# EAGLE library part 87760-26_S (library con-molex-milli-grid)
HEADER
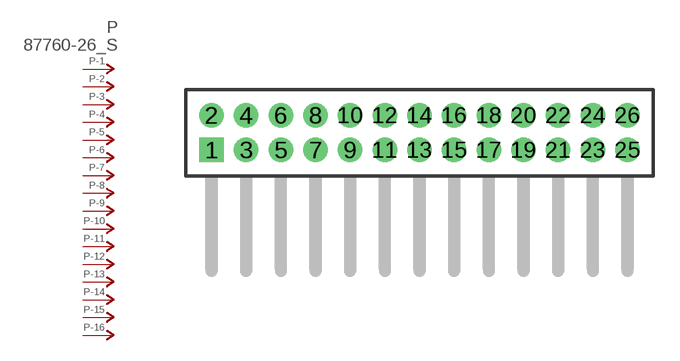
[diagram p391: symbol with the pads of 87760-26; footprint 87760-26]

Designator prefix P; gates -1=P-NV -2=P-N -3=P-N -4=P-N -5=P-N -6=P-N -7=P-N -8=P-N -9=P-N -10=P-N -11=P-N -12=P-N -13=P-N -14=P-N -15=P-N -16=P-N -17=P-N -18=P-N -19=P-N -20=P-N -21=P-N -22=P-N -23=P-N -24=P-N -25=P-N -26=P-N

## 87760-26_S  [87760-26]
1  -1:P  pas
2  -2:P  pas
3  -3:P  pas
4  -4:P  pas
5  -5:P  pas
6  -6:P  pas
7  -7:P  pas
8  -8:P  pas
9  -9:P  pas
10  -10:P  pas
11  -11:P  pas
12  -12:P  pas
13  -13:P  pas
14  -14:P  pas
15  -15:P  pas
16  -16:P  pas
17  -17:P  pas
18  -18:P  pas
19  -19:P  pas
20  -20:P  pas
21  -21:P  pas
22  -22:P  pas
23  -23:P  pas
24  -24:P  pas
25  -25:P  pas
26  -26:P  pas

## Footprint 87760-26 (pad centres in mm)
HEADER Dual Row, Right Angle
drill 0.914 square: 1 -12,-1
drill 0.914: 2 -12,1; 3 -10,-1; 4 -10,1; 5 -8,-1; 6 -8,1; 7 -6,-1; 8 -6,1; 9 -4,-1; 10 -4,1; 11 -2,-1; 12 -2,1; 13 0,-1; 14 0,1; 15 2,-1; 16 2,1; 17 4,-1; 18 4,1; 19 6,-1; 20 6,1; 21 8,-1; 22 8,1; 23 10,-1; 24 10,1; 25 12,-1; 26 12,1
